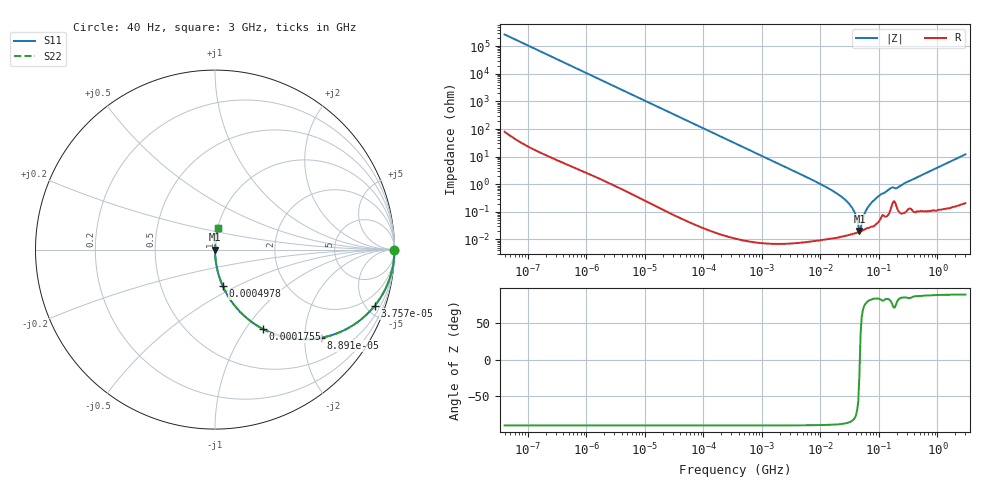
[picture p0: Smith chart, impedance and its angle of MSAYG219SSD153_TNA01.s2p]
! MSAYG219SSD153_TNA01  S-PARAMETER MODEL  ( General Type )
! Model Generated by TAIYO YUDEN Corporation (http://www.ty-top.com)
! Version 2.0
! TAIYO YUDEN Control No. 031016
! Copyright(c) 2003 TAIYO YUDEN CO.,LTD. All Rights Reserved.
! Product Description (link to TY-COMPAS)
! https://ds.yuden.co.jp/TYCOMPAS/or/detail?pn=MSAYG219SSD153KTNA01&u=M
! Products Name : Multilayer Ceramic Capacitors
! Characteristics :
!  Capacitance : 0.015 uF , Rated Voltage : 35V
!  Case Size : 2.0 x 1.25 / 0.079 x 0.049 [mm/inch] , Thickness : 0.85 / 0.033 [mm/inch]
!  (Conditions: Temperature = 25 degC , DC Bias Current/Voltage = 0A / 0V)
! External Node Assignments :
!  1  o---| |---o  2
! GND o---------o GND
! Frequency Range : 40Hz  -  3GHz  [ 401 STEP ]
# MHz S RI R 50
! Freq[MHz].  S11 Real  S11 Imag  S21 Real  S21 Imag  S12 Real  S12 Imag  S22 Real  S22 Imag
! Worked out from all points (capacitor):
!   401 points, 40 Hz to 3 GHz, reference 50 ohm
!   read as one part in series: C = 14.9 nF near 44 Hz
!   lowest |Z| = 20.2 mohm at 46.33 MHz (marker M1)
!   series resonance near 47.09 MHz, so ESL is about 760 pH
!   S11 on the Smith chart (normalised r, x): 40 Hz: open; 37.58 kHz: 1.00, -5.67; 88.91 kHz: 1.00, -2.40; 175.5 kHz: 1.00, -1.21; 497.8 kHz: 1.00, -0.43; 3 GHz: 1.00, +0.24
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4e-05  1 -0.000376  2.53e-07 0.000376  2.53e-07 0.000376  1 -0.000376
0.000834  0.9999 -0.00783  6.32e-05 0.00783  6.32e-05 0.00783  0.9999 -0.00783
0.00535  0.9975 -0.0501  0.00253 0.0501  0.00253 0.0501  0.9975 -0.0501
0.017386  0.974 -0.159  0.026 0.159  0.026 0.159  0.974 -0.159
0.037575  0.8892 -0.3137  0.1108 0.3137  0.1108 0.3137  0.8892 -0.3137
0.088912  0.5892 -0.4919  0.4108 0.4919  0.4108 0.4919  0.5892 -0.4919
0.175499  0.2692 -0.4434  0.7308 0.4434  0.7308 0.4434  0.2692 -0.4434
0.362475  0.0795 -0.2704  0.9205 0.2704  0.9205 0.2704  0.0795 -0.2704
0.497842  0.0438 -0.2045  0.9562 0.2045  0.9562 0.2045  0.0438 -0.2045
1.477731  0.00522 -0.0716  0.9948 0.0716  0.9948 0.0716  0.00522 -0.0716
7.222098  0.000293 -0.0144  0.9997 0.0144  0.9997 0.0144  0.000293 -0.0144
17.08948  0.00014 -0.0054  0.9999 0.0054  0.9999 0.0054  0.00014 -0.0054
26.8909  0.000143 -0.00265  0.9999 0.00265  0.9999 0.00265  0.000143 -0.00265
35.29647  0.000159 -0.00132  0.9998 0.00132  0.9998 0.00132  0.000159 -0.00132
46.32945  0.000189 -7.29e-05  0.9998 7.29e-05  0.9998 7.29e-05  0.000189 -7.29e-05
50.72622  0.000204 0.000331  0.9998 -0.000331  0.9998 -0.000331  0.000204 0.000331
58.11596  0.000237 0.000941  0.9998 -0.000941  0.9998 -0.000941  0.000237 0.000941
69.67004  0.000272 0.00178  0.9997 -0.00178  0.9997 -0.00178  0.000272 0.00178
95.68847  0.000416 0.0035  0.9996 -0.0035  0.9996 -0.0035  0.000416 0.0035
150.5692  0.000975 0.00657  0.999 -0.00657  0.999 -0.00657  0.000975 0.00657
206.7996  0.00131 0.00735  0.9987 -0.00735  0.9987 -0.00735  0.00131 0.00735
3000  0.0163 0.1185  0.9837 -0.1185  0.9837 -0.1185  0.0163 0.1185
